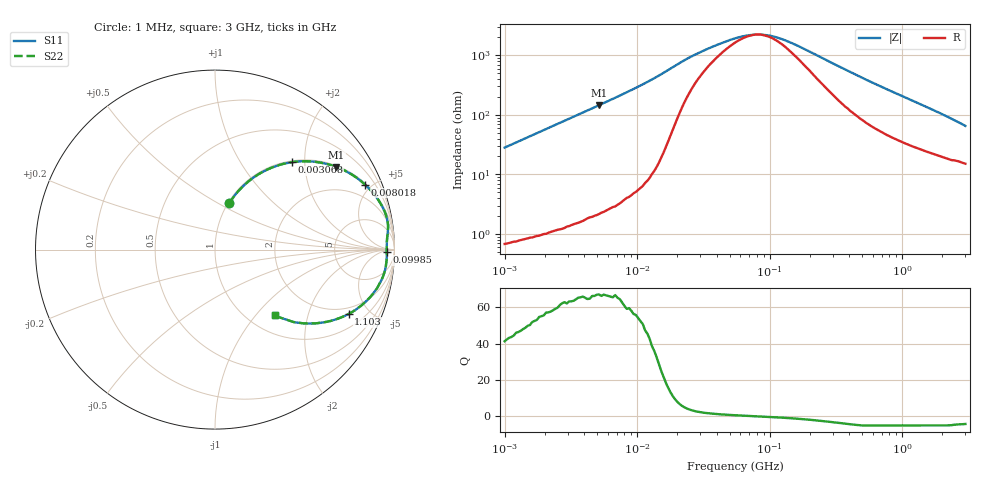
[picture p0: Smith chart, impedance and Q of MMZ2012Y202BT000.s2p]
! S-parameter Generated by TDK Corporation
! Copyright(C) 2016 TDK Corporation.
! All Rights Reserved.
! TDK P/N: MMZ2012Y202BT000 (Chip Beads)
! Property: |Z|=2000¶ at 100MHz
! Size(LxWxT): 2x1.25x0.85mm, 0.079x0.049x0.033inches
! Model Type: s2p (Touchstone File Format Version 1.0)
! Frequency: DC=Yes Start=1MHz Stop=3000MHz 202points Log-sweep
! Note: This model was converted from impedance.
! Model Generated on May. 16, 2016
! Hash(MD5):
! Port Assignments:
!  1 ---@@@--- 2
! Applicable Conditions:
!  Temperature = 25 degC
!  DC Bias Current = 0 A
!  Small Signal Operation
! Terms and conditions regarding TDK Simulation Models
! (1)This simulation model is being provided solely for informational purposes. Please refer to the specifications of the products in terms of detailed characteristics of such products.
! (2)In no event shall TDK Corporation of any of its subsidiaries be liable for any loss or damage arising, directly or indirectly,
!  From any information contained in this simulation model, including, but not limited to loss or damages arising from any inaccuracies, omissions or errors in connection with such information.
! (3)Any and all copyrights on this simulation model are owned by TDK Corporation.
!  Duplication or redistribution of this simulation model without prior written permission from TDK Corporation is prohibited.
! (4)This simulation model is subject to any modification or change without any prior notice.
! (5)Neither TDK Corporation nor any of its subsidiaries shall make any warranty, express or implied,
!  Including but not limited to the correctness, implied warranties of merchantability and fitness for a particular purpose with respect to this simulation models.
! (6)The use of this simulation model shall be deemed to have consented to the terms and conditions hereof.
# MHz S MA R 50
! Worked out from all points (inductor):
!   201 points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, 1 MHz to 3 GHz, reference 50 ohm
!   read as one part in series: L = 4.48 uH near 1.041 MHz
!   highest Q = 67 at 5.162 MHz (marker M1), where L = 4.48 uH
!   self-resonance near 81.13 MHz
!   S11 on the Smith chart (normalised r, x): 1 MHz: 1.01, +0.56; 3.068 MHz: 1.03, +1.72; 8.018 MHz: 1.08, +4.58; 99.85 MHz: 42, -13; 1.103 GHz: 1.63, -3.70; 3 GHz: 1.30, -1.27
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1  0.2696 73.0  0.9565 -15.6  0.9565 -15.6  0.2696 73.0
1.323425  0.3467 68.5  0.9306 -20.3  0.9306 -20.3  0.3467 68.5
1.751453  0.4383 62.9  0.8906 -26.0  0.8906 -26.0  0.4383 62.9
2.317916  0.5408 56.3  0.8319 -32.7  0.8319 -32.7  0.5408 56.3
3.067588  0.647 48.8  0.7524 -40.3  0.7524 -40.3  0.647 48.8
3.900413  0.7325 42.0  0.6698 -47.1  0.6698 -47.1  0.7325 42.0
5.161903  0.8179 34.3  0.5633 -54.9  0.5633 -54.9  0.8179 34.3
8.017732  0.9111 23.4  0.3976 -65.6  0.3976 -65.6  0.9111 23.4
10.61086  0.9468 17.7  0.3043 -71.2  0.3043 -71.2  0.9468 17.7
14.61624  0.9699 12.2  0.2122 -75.8  0.2122 -75.8  0.9699 12.2
27.73354  0.9648 5.0  0.09274 -65.2  0.09274 -65.2  0.9648 5.0
39.76269  0.9591 2.9  0.06459 -49.2  0.06459 -49.2  0.9591 2.9
54.77226  0.9574 1.5  0.04981 -30.5  0.04981 -30.5  0.9574 1.5
75.44761  0.9572 0.3  0.04309 -6.4  0.04309 -6.4  0.9572 0.3
99.84923  0.9574 -0.8  0.04473 17.4  0.04473 17.4  0.9574 -0.8
137.5402  0.958 -2.2  0.05602 40.3  0.05602 40.3  0.958 -2.2
213.6344  0.9576 -4.6  0.08915 59.4  0.08915 59.4  0.9576 -4.6
457.0858  0.9378 -11.5  0.2037 66.6  0.2037 66.6  0.9378 -11.5
800.5644  0.8829 -19.7  0.3426 60.5  0.3426 60.5  0.8829 -19.7
1102.76  0.8263 -25.7  0.4405 54.5  0.4405 54.5  0.8263 -25.7
1931.433  0.6693 -38.0  0.6267 41.1  0.6267 41.1  0.6693 -38.0
3000  0.4959 -47.7  0.7609 28.8  0.7609 28.8  0.4959 -47.7
